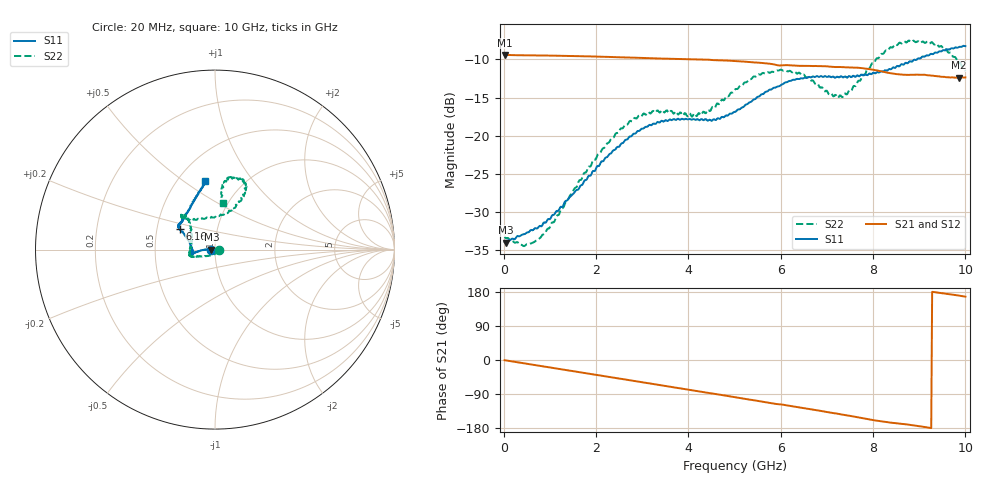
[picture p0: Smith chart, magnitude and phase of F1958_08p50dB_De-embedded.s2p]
! Integrated Device Technology
! Corporate Headquarters
! 6024 Silver Creek Valley Road
! San Jose, CA 95138  USA
! Phone:  1-408-284-8200
! Toll Free:  1-800-223-1366
! Webpage:  http://www.idt.com/
! Timing and RF Division
! 515 Groton Road, Suite 102
! Westford, MA 01886-6024
! Device:  F1958
! Description: 7-bit 0.25 dB Digital Step Attenuator
! Frequency:  0.001 -  6.000 GHz
! Package:  4x4 mm Thin QFN Plastic Package: 24 pin
! Ports:  2 RF, 12 DC
!  Pin  1  = D0
!  Pin  2  = VDD
!  Pin  3  = VMODE
!  Pin  4  = GND
!  Pin  5  = RF1  =  Port 1
!  Pin  6  = GND
!  Pin  7  = GND
!  Pin  8  = GND
!  Pin  9  = GND
!  Pin 10  = GND
!  Pin 11  = GND
!  Pin 12  = GND
!  Pin 13  = GND
!  Pin 14  = RF2  =  Port 2
!  Pin 15  = GND
!  Pin 16  = LE
!  Pin 17  = CLK
!  Pin 18  = DATA
!  Pin 19  = D6
!  Pin 20  = D5
!  Pin 21  = D4
!  Pin 22  = D3
!  Pin 23  = D2
!  Pin 24  = D1
! State:  34
! Atten State:  8.50 dB
! Voltage:  +3.30 Volts
! Current:  0.258 mA
! Data:  The device was measured on a F1958 evaluation board which has
!  individual transmission lines to the RF pins.  Data was collected
!  using a calibrated network analyzer.  The evaluation board was
!  de-embedded using Automatic Fixture Removal (AFR).
!  The reference plane is the edge of the package pin.
! Misc:
!  Action Tracker AT0419
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# GHz S dB R 50
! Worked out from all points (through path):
!   500 points, 20 MHz to 10 GHz, reference 50 ohm
!   highest |S21| = -9.39 dB at 20 MHz (marker M1); lowest = -12.4 dB at 9.86 GHz (marker M2)
!   group delay of S21, straight-line fit = 54.1 ps
!   lowest |S11| = -34.1 dB at 40 MHz (marker M3), VSWR 1.04, Z = 48.1 - j0.0797 ohm
!   |S11| at or under -10 dB: start of sweep to 8.949 GHz
!   |S22| runs from -34.5 to -7.5 dB; largest |S21 - S12| = 0.001
!   S11 on the Smith chart (normalised r, x): 20 MHz: 0.96, -0.00; 6.16 GHz: 0.66, +0.16; 10 GHz: 0.67, +0.60
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0.02  -34.01 -177.7  -9.39 -0.5  -9.39 -0.5  -33.26 -5.9
0.04  -34.06 -177.6  -9.40 -0.9  -9.40 -0.9  -33.45 -9.1
0.42  -32.98 175.6  -9.45 -8.4  -9.45 -8.3  -34.49 -36.6
0.76  -31.97 175.6  -9.47 -15.0  -9.47 -15.0  -33.59 -69.6
1.1  -30.35 177.7  -9.50 -21.6  -9.50 -21.6  -31.28 -102.2
1.7  -26.49 -179.4  -9.58 -33.3  -9.57 -33.3  -25.55 -139.6
2.58  -20.99 -173.7  -9.72 -50.5  -9.71 -50.5  -19.04 -159.6
2.92  -19.39 -171.7  -9.78 -57.1  -9.77 -57.2  -17.40 -163.4
3.36  -18.27 -169.6  -9.87 -65.7  -9.87 -65.8  -16.87 -166.5
4.24  -17.99 -173.8  -10.00 -82.8  -10.01 -82.9  -17.07 164.5
5.02  -16.88 166.5  -10.20 -98.3  -10.21 -98.3  -13.89 134.6
5.54  -14.84 155.2  -10.43 -108.6  -10.44 -108.6  -11.98 131.7
6.16  -12.90 150.0  -10.75 -120.2  -10.76 -120.2  -11.57 134.8
6.68  -12.27 146.9  -10.86 -130.3  -10.87 -130.2  -12.75 131.0
7.1  -12.33 142.8  -10.96 -139.4  -10.97 -139.3  -14.47 112.3
7.34  -12.34 141.4  -11.01 -144.2  -11.01 -144.1  -14.95 91.5
7.9  -11.94 130.1  -11.24 -156.3  -11.24 -156.4  -11.19 65.2
8.34  -11.28 120.5  -11.77 -164.7  -11.77 -164.8  -8.69 62.3
8.76  -10.46 111.7  -12.03 -170.5  -12.03 -170.4  -7.55 67.5
9.26  -9.26 103.8  -12.12 -179.7  -12.12 -179.8  -7.74 78.1
9.86  -8.36 98.6  -12.39 170.0  -12.42 170.1  -10.35 82.3
10  -8.25 98.6  -12.35 167.1  -12.38 167.2  -11.53 80.7
